| TEXAS INSTRUMENTS INCORPORATED
| Standard Linear and Logic Group
| IBIS Model of PCF8574
| REMOTE 8-BIT I/O EXPANDER FOR I2C BUS
| This file contains package information for the following:
|  SOIC 16-pin (DW) package as [Component] PCF8574_DW
|  PDIP 16-pin (N) package as [Component] PCF8574_N
|  TSSOP 20-pin (PW) package as [Component] PCF8574_PW
|  TVSOP 20-pin (DGV) package as [Component] PCF8574_DGV
|  QFN 20-pin (RGY) package as [Component] PCF8574_RGY
| This device can be powered at the following Vccs:
|  6 volt Vcc
|  2.5 volt Vcc
| This file provides unique models under the [Model Selector] for each Vcc.
| For operation at a specific Vcc, select the appropriate model after each
| [Model Selector] keyword.
[IBIS Ver]   3.2
[Comment char]  |_char
[File Name]   pcf8574.ibs
[File Rev]   1.1 | x_die
[Date]   October 21, 2005
[Source]   Data created from TI-SPICE simulations at TI-SLL.
[Notes]   The following is an IBIS list for the PCF8574.
   Please contact sllibis@ti.com with questions and
   comments concerning SLL IBIS models.
   - FILE REV HISTORY
   - 1.1 Release IBIS file on 10/21/05
   - End point warning due to AC and DC mismatch.
   - Power clamp data has been deleted in all models except
   I/O models as there is no power-clamp diode.
   - Non-monotonic data due to FET characteristics.
[Disclaimer] Property of Texas Instruments Incorporated.  Unauthorized
   reproduction and/or distribution is strictly prohibited.
   This product is protected under copyright law.
   Created  2005, (C) Copyright  2005, Texas Instruments
   Incorporated, All Rights Reserved
   UNLESS THERE IS A SIGNED, WRITTEN AGREEMENT TO THE
   CONTRARY, TEXAS INSTRUMENTS (TI) IS PROVIDING THE IBIS
   MODELS  AND WITHOUT ANY WARRANTY, EXPRESSED OR
   IMPLIED.  TI assumes no liability for:
   1) the accuracy of the IBIS models provided to your
   company;
   2) the proper functioning of these IBIS Models in your
   design or for any resulting applications; or
   3) infringement of patents, copyrights or intellectual
   property rights resulting from your use of these IBIS
   models.
   TI provides IBIS Models as a service to our customers.
   You and your company shall not distribute, sell or give
   these models to anyone else without prior written
   permission from TI.
   TI reserves the right to make changes to our products or
   to discontinue any semiconductor product or service
   without notice, and advises our customers to obtain the
   latest version of relevant information to verify, before
   placing orders, that the information being relied on is
   current.
   Please be aware that your receipt and use of the IBIS
   information provided shall serve as acceptance of these
   terms and conditions.  If you do not accept these terms,
   you should return or destroy the IBIS models and any
   other accompanying information immediately.
| Component PCF8574_DW 16-pin SOIC
[Component]   PCF8574_DW
[Manufacturer]   Texas Instruments, Inc.
[Package]
|   typ   min   max
R_pkg   4.600e-02   3.400e-02   5.700e-02
L_pkg   4.858e-09   3.987e-09   6.214e-09
C_pkg   7.150e-13   5.020e-13   1.046e-12
[Pin]   signal_name   model_name   R_pin   L_pin   C_pin
1   A0   PCF8574_A   5.700e-02   6.214e-09   1.026e-12
2   A1   PCF8574_A   5.500e-02   5.236e-09   8.180e-13
3   A2   PCF8574_A   3.400e-02   3.987e-09   7.230e-13
4   P0   PCF8574_P   3.600e-02   3.996e-09   7.260e-13
5   P1   PCF8574_P   3.600e-02   3.996e-09   7.260e-13
6   P2   PCF8574_P   3.400e-02   3.987e-09   7.040e-13
7   P3   PCF8574_P   5.500e-02   5.236e-09   8.180e-13
8   GND   GND   5.700e-02   6.214e-09   1.046e-12
9   P4   PCF8574_P   5.700e-02   6.214e-09   8.270e-13
10   P5   PCF8574_P   5.500e-02   5.236e-09   5.970e-13
11   P6   PCF8574_P   3.400e-02   3.987e-09   5.020e-13
12   P7   PCF8574_P   3.600e-02   3.996e-09   5.050e-13
13   INTZ   PCF8574_INTZ   3.600e-02   3.996e-09   5.050e-13
14   SCL   PCF8574_SCL   3.400e-02   3.987e-09   5.020e-13
15   SDA   PCF8574_SDA   5.500e-02   5.236e-09   5.970e-13
16   VCC   POWER   5.700e-02   6.214e-09   8.270e-13
| Component PCF8574_N 16-pin PDIP
[Component]   PCF8574_N
[Manufacturer]   Texas Instruments, Inc.
[Package]
|   typ   min   max
R_pkg   5.600e-02   5.200e-02   6.300e-02
L_pkg   7.637e-09   5.451e-09   1.053e-08
C_pkg   5.280e-13   3.350e-13   8.930e-13
[Pin]   signal_name   model_name   R_pin   L_pin   C_pin
1   A0   PCF8574_A   5.800e-02   1.053e-08   8.920e-13
2   A1   PCF8574_A   6.200e-02   8.759e-09   5.350e-13
3   A2   PCF8574_A   5.200e-02   7.146e-09   3.870e-13
4   P0   PCF8574_P   5.300e-02   5.451e-09   4.080e-13
5   P1   PCF8574_P   5.300e-02   5.513e-09   3.700e-13
6   P2   PCF8574_P   5.300e-02   6.304e-09   3.360e-13
7   P3   PCF8574_P   5.700e-02   7.830e-09   5.030e-13
8   GND   GND   5.600e-02   9.581e-09   8.050e-13
9   P4   PCF8574_P   5.800e-02   9.603e-09   8.070e-13
10   P5   PCF8574_P   6.200e-02   7.864e-09   5.030e-13
11   P6   PCF8574_P   5.200e-02   6.295e-09   3.350e-13
12   P7   PCF8574_P   5.300e-02   5.499e-09   3.560e-13
13   INTZ   PCF8574_INTZ   5.300e-02   5.452e-09   4.040e-13
14   SCL   PCF8574_SCL   5.300e-02   7.156e-09   3.870e-13
15   SDA   PCF8574_SDA   6.300e-02   8.740e-09   5.340e-13
16   VCC   POWER   5.600e-02   1.048e-08   8.930e-13
| Component PCF8574_PW 20-pin TSSOP
[Component]   PCF8574_PW
[Manufacturer]   Texas Instruments, Inc.
[Package]
|   typ   min   max
R_pkg   5.000e-02   4.200e-02   6.000e-02
L_pkg   2.802e-09   2.248e-09   3.553e-09
C_pkg   3.170e-13   2.020e-13   4.430e-13
[Pin]   signal_name   model_name   R_pin   L_pin   C_pin
1   INTZ   PCF8574_INTZ   5.500e-02   3.461e-09   4.400e-13
2   SCL   PCF8574_SCL   5.500e-02   3.150e-09   4.010e-13
3   NC   NC   4.200e-02   2.619e-09   3.020e-13
4   SDA   PCF8574_SDA   4.500e-02   2.273e-09   2.020e-13
5   VCC   POWER   4.500e-02   2.248e-09   2.240e-13
6   A0   PCF8574_A   4.500e-02   2.273e-09   2.260e-13
7   A1   PCF8574_A   4.400e-02   2.323e-09   2.050e-13
8   NC   NC   4.600e-02   2.704e-09   3.070e-13
9   A2   PCF8574_A   6.000e-02   3.265e-09   4.110e-13
10   P0   PCF8574_P   5.700e-02   3.506e-09   4.360e-13
11   P1   PCF8574_P   5.800e-02   3.553e-09   4.370e-13
12   P2   PCF8574_P   5.800e-02   3.193e-09   4.050e-13
13   NC   NC   4.200e-02   2.704e-09   3.110e-13
14   P3   PCF8574_P   4.600e-02   2.392e-09   2.100e-13
15   GND   GND   4.700e-02   2.334e-09   2.290e-13
16   P4   PCF8574_P   4.700e-02   2.300e-09   2.270e-13
17   P5   PCF8574_P   4.700e-02   2.349e-09   2.070e-13
18   NC   NC   4.500e-02   2.677e-09   3.060e-13
19   P6   PCF8574_P   6.000e-02   3.235e-09   4.060e-13
20   P7   PCF8574_P   5.600e-02   3.487e-09   4.430e-13
| Component PCF8574_DGV 20-pin TVSOP
[Component]   PCF8574_DGV
[Manufacturer]   Texas Instruments, Inc.
[Package]
|   typ   min   max
R_pkg   4.400e-02   3.800e-02   4.800e-02
L_pkg   2.561e-09   2.236e-09   2.961e-09
C_pkg   3.420e-13   2.640e-13   4.460e-13
[Pin]   signal_name   model_name   R_pin   L_pin   C_pin
1   INTZ   PCF8574_INTZ   4.400e-02   2.935e-09   4.170e-13
2   SCL   PCF8574_SCL   4.200e-02   2.869e-09   4.460e-13
3   NC   NC   4.300e-02   2.399e-09   3.160e-13
4   SDA   PCF8574_SDA   4.400e-02   2.236e-09   2.650e-13
5   VCC   POWER   4.600e-02   2.278e-09   2.640e-13
6   A0   PCF8574_A   4.500e-02   2.274e-09   2.640e-13
7   A1   PCF8574_A   4.400e-02   2.285e-09   2.690e-13
8   NC   NC   4.300e-02   2.452e-09   3.200e-13
9   A2   PCF8574_A   4.400e-02   2.900e-09   4.460e-13
10   P0   PCF8574_P   4.400e-02   2.961e-09   4.180e-13
11   P1   PCF8574_P   4.500e-02   2.954e-09   4.180e-13
12   P2   PCF8574_P   4.200e-02   2.847e-09   4.430e-13
13   NC   NC   4.500e-02   2.453e-09   3.190e-13
14   P3   PCF8574_P   4.500e-02   2.297e-09   2.690e-13
15   GND   GND   4.800e-02   2.334e-09   2.680e-13
16   P4   PCF8574_P   4.800e-02   2.335e-09   2.670e-13
17   P5   PCF8574_P   4.600e-02   2.299e-09   2.680e-13
18   NC   NC   4.600e-02   2.457e-09   3.200e-13
19   P6   PCF8574_P   4.300e-02   2.848e-09   4.410e-13
20   P7   PCF8574_P   3.800e-02   2.812e-09   4.080e-13
| Component PCF8574_RGY 20-pin QFN
[Component]   PCF8574_RGY
[Manufacturer]   Texas Instruments, Inc.
[Package]
|   typ   min   max
R_pkg   5.000e-02   4.600e-02   5.500e-02
L_pkg   1.119e-09   1.025e-09   1.227e-09
C_pkg   3.520e-13   3.440e-13   3.630e-13
[Pin]   signal_name   model_name   R_pin   L_pin   C_pin
1   INTZ   PCF8574_INTZ   5.200e-02   1.167e-09   3.600e-13
2   SCL   PCF8574_SCL   4.700e-02   1.049e-09   3.440e-13
3   NC   NC   4.700e-02   1.055e-09   3.450e-13
4   SDA   PCF8574_SDA   5.000e-02   1.119e-09   3.500e-13
5   VCC   POWER   5.500e-02   1.227e-09   3.600e-13
6   A0   PCF8574_A   5.200e-02   1.167e-09   3.550e-13
7   A1   PCF8574_A   4.900e-02   1.087e-09   3.480e-13
8   NC   NC   4.700e-02   1.054e-09   3.460e-13
9   A2   PCF8574_A   4.900e-02   1.091e-09   3.490e-13
10   P0   PCF8574_P   5.300e-02   1.184e-09   3.620e-13
11   P1   PCF8574_P   5.300e-02   1.181e-09   3.600e-13
12   P2   PCF8574_P   5.000e-02   1.108e-09   3.490e-13
13   NC   NC   4.800e-02   1.075e-09   3.470e-13
14   P3   PCF8574_P   5.000e-02   1.107e-09   3.490e-13
15   GND   GND   5.400e-02   1.200e-09   3.620e-13
16   P4   PCF8574_P   5.100e-02   1.141e-09   3.570e-13
17   P5   PCF8574_P   4.700e-02   1.043e-09   3.440e-13
18   NC   NC   4.600e-02   1.025e-09   3.440e-13
19   P6   PCF8574_P   4.900e-02   1.090e-09   3.490e-13
20   P7   PCF8574_P   5.400e-02   1.204e-09   3.630e-13
| Model PCF8574_SCL
[Model Selector]   PCF8574_SCL
PCF8574_SCL_60   6 volt Vcc
PCF8574_SCL_25B   2.5 volt Vcc
| Model PCF8574_A
[Model Selector]   PCF8574_A
PCF8574_A_60   6 volt Vcc
PCF8574_A_25B   2.5 volt Vcc
| Model PCF8574_SDA
[Model Selector]   PCF8574_SDA
PCF8574_SDA_60   6 volt Vcc
PCF8574_SDA_25B   2.5 volt Vcc
| Model PCF8574_P
[Model Selector]   PCF8574_P
PCF8574_P_60   6 volt Vcc
PCF8574_P_25B   2.5 volt Vcc
| Model PCF8574_INTZ
[Model Selector]   PCF8574_INTZ
PCF8574_INTZ_60   6 volt Vcc
PCF8574_INTZ_25B   2.5 volt Vcc
| Models and submodels in the file (10): PCF8574_SCL_60 (Input), PCF8574_SCL_25B (Input), PCF8574_A_60 (Input), PCF8574_A_25B (Input), PCF8574_SDA_60 (I/O_open_drain), PCF8574_SDA_25B (I/O_open_drain), PCF8574_P_60 (I/O_open_drain), PCF8574_P_25B (I/O_open_drain), PCF8574_INTZ_60 (Open_drain), PCF8574_INTZ_25B (Open_drain)
